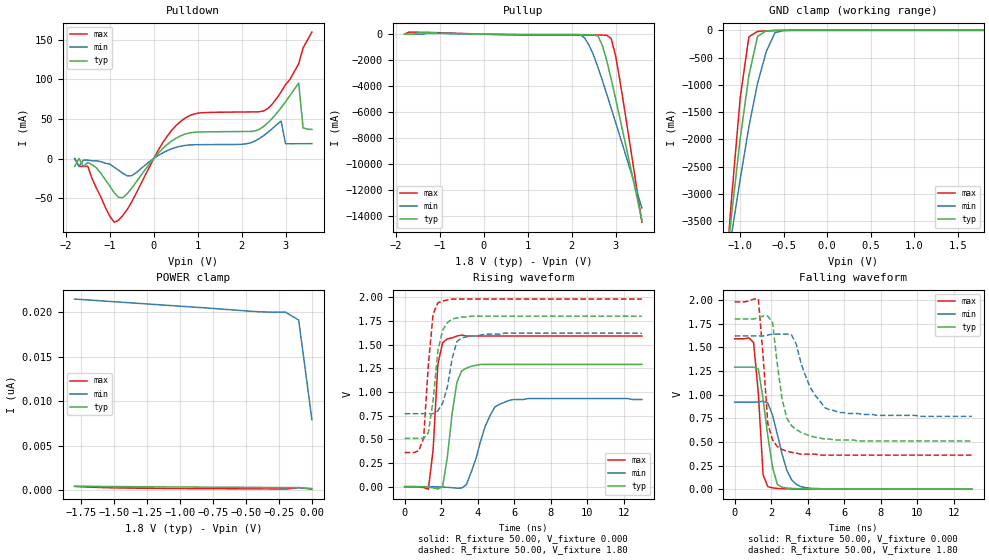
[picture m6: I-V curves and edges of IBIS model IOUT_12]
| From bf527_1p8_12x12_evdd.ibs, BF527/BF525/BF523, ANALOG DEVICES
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|   Model prw0812swcdg_25
[Model]   IOUT_12
Model_type   I/O
Polarity   Non-Inverting
Enable   Active-Low
Vinl =   0.70V
Vinh =   1.00V
Vmeas =   1.20V
Cref =  50.00pF
Rref =   1.00M
Vref =  0.000V
C_comp   4.32pF   3.89pF   4.75pF
[Temperature Range]   25.00   0.12k   -40.00
[Voltage Range]   1.80V   1.62V   1.98V
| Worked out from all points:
|   slope of the pulldown table from 0 to 0.27 V, typ, clamps not added: 17 ohm
|   slope of the pullup table from 0 to 0.27 V, typ, clamps not added: 16.9 ohm
|   GND clamp passes 1 mA (typ) near -0.53 V on its own axis
|   rising waveform, R_fixture 50.00, V_fixture 0.000: 20-80 % time 510ps typ, 944ps min, 300ps max; typ from 0 V to 1.29 V
|   rising waveform, R_fixture 50.00, V_fixture 1.80: 20-80 % time 501ps typ, 573ps min, 382ps max; typ from 0.51 V to 1.8 V
|   falling waveform, R_fixture 50.00, V_fixture 0.000: 20-80 % time 565ps typ, 764ps min, 335ps max; typ from 1.29 V to 0 V
|   falling waveform, R_fixture 50.00, V_fixture 1.80: 20-80 % time 628ps typ, 1.15ns min, 376ps max; typ from 1.8 V to 0.51 V
[Pulldown]
| voltage   I(typ)   I(min)   I(max)
-1.8V     -10mA      0A         0A
-1.4V     -8mA       -3mA       -26mA
-1V       -35mA      -7mA       -73mA
-800mV    -49.2mA    -14.8mA    -78.14mA
-500mV    -37.44mA   -21.82mA   -54.81mA
600mV     28.34mA    15.42mA    46.41mA
2.5V      40.54mA    28.91mA    60.13mA
2.9V      64.32mA    47.33mA    84.42mA
3V        71.81mA    18.78mA    93.51mA
3.3V      95.51mA    18.69mA    120mA
3.4V      38.66mA    18.74mA    140mA
3.6V      36.76mA    18.88mA    160mA
[Pullup]
| voltage   I(typ)   I(min)   I(max)
-1.8V     1.83mA     550uA      15.88mA
-1.6V     4.2mA      570uA      160mA
2.2V      -36.14mA   -47.43mA   -60.12mA
2.3V      -36.65mA   -310mA     -60.23mA
2.4V      -38.95mA   -860mA     -60.39mA
2.6V      -150mA     -2.55A     -65.28mA
2.7V      -860mA     -3.56A     -72.48mA
2.8V      -2.03A     -4.61A     -83.95mA
2.9V      -3.44A     -5.68A     -330mA
3V        -4.94A     -6.77A     -1.64A
3.1V      -6.47A     -7.85A     -3.57A
3.6V      -14.32A    -13.36A    -14.46A
[GND_clamp]
| voltage   I(typ)   I(min)   I(max)
-1.8V     -14.28A    -11.35A    -18.41A
-1.2V     -4.9A      -4.81A     -5.19A
-1.1V     -3.4A      -3.75A     -3.1A
-1V       -1.99A     -2.73A     -1.24A
-900mV    -830mA     -1.77A     -120mA
-800mV    -110mA     -970mA     -19.21mA
-700mV    -9.89mA    -390mA     -9.78mA
-600mV    -2.57mA    -42.87mA   -3.5mA
-500mV    -460uA     -4.38mA    -550uA
1.8V      170pA      19.94nA    82.46pA
[POWER_clamp]
| voltage   I(typ)   I(min)   I(max)
-1.8V     440pA      21.46nA    400pA
-1.3V     370pA      20.96nA    200pA
-400mV    290pA      20.03nA    130pA
-200mV    270pA      19.99nA    110pA
-100mV    270pA      19.09nA    270pA
0V        170pA      7.92nA     95.65pA
[Ramp]
| variable   typ   min   max
dV/dt_r   0.78/0.48n   0.55/0.89n   0.96/0.28n
dV/dt_f   0.77/0.58n   0.51/1.05n   0.97/0.32n
R_load = 50.00
[Rising Waveform]
R_fixture = 50.00
V_fixture = 0.000
V_fixture_min = 0.000
V_fixture_max = 0.000
L_fixture = 0.000H
C_fixture = 0.000F
| time   V(typ)   V(min)   V(max)
0s        0V         0V         0V
1.3ns     -5.63mV    48.64uV    -26.39mV
1.56ns    -11.11mV   -580uV     390mV
1.82ns    -24.52mV   -2.73mV    1.29V
2.08ns    -100uV     -5.1mV     1.52V
2.34ns    310mV      -6.78mV    1.56V
2.86ns    1.1V       -15.45mV   1.59V
3.38ns    1.25V      19.11mV    1.59V
5.2ns     1.29V      870mV      1.59V
13ns      1.29V      920mV      1.59V
[Rising Waveform]
R_fixture = 50.00
V_fixture = 1.80
V_fixture_min = 1.62
V_fixture_max = 1.98
L_fixture = 0.000H
C_fixture = 0.000F
| time   V(typ)   V(min)   V(max)
0s        510mV      770mV      360mV
780ps     510mV      770mV      380mV
1.04ns    510mV      770mV      510mV
1.3ns     570mV      770mV      1.29V
1.56ns    910mV      770mV      1.82V
1.82ns    1.43V      800mV      1.94V
2.34ns    1.73V      1.05V      1.97V
2.86ns    1.78V      1.53V      1.98V
3.12ns    1.79V      1.57V      1.98V
13ns      1.8V       1.62V      1.98V
[Falling Waveform]
R_fixture = 50.00
V_fixture = 0.000
V_fixture_min = 0.000
V_fixture_max = 0.000
L_fixture = 0.000H
C_fixture = 0.000F
| time   V(typ)   V(min)   V(max)
0s        1.29V      920mV      1.59V
1.04ns    1.29V      920mV      1.55V
1.3ns     1.27V      920mV      1.01V
1.56ns    950mV      930mV      150mV
1.82ns    560mV      910mV      26.05mV
2.08ns    230mV      780mV      13.64mV
2.34ns    50.45mV    580mV      8.12mV
2.86ns    12.62mV    200mV      3.96mV
3.64ns    4.08mV     25.47mV    1.23mV
13ns      -7.47uV    -14.21uV   -16.13uV
[Falling Waveform]
R_fixture = 50.00
V_fixture = 1.80
V_fixture_min = 1.62
V_fixture_max = 1.98
L_fixture = 0.000H
C_fixture = 0.000F
| time   V(typ)   V(min)   V(max)
0s        1.8V       1.62V      1.98V
1.3ns     1.81V      1.62V      2.01V
1.82ns    1.83V      1.63V      690mV
2.08ns    1.76V      1.64V      520mV
2.34ns    1.32V      1.64V      450mV
2.86ns    750mV      1.64V      400mV
3.38ns    630mV      1.53V      380mV
4.16ns    560mV      1.07V      370mV
5.72ns    520mV      810mV      360mV
13ns      510mV      770mV      360mV
